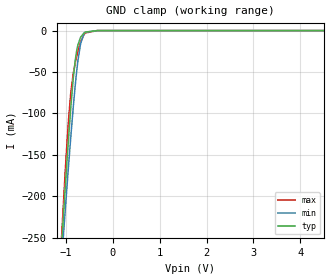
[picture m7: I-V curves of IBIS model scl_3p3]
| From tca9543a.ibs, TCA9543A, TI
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|   scl_3p3 Model
[Model]   scl_3p3
Model_type   Input
Vinl = 0.99
Vinh = 2.31
|   typ   min   max
|   (nom PVT)   (fast PVT)   (slow PVT)
C_comp   7.826e-12   4.224e-12   1.127e-11
[Model spec]
|subparameter
Vinl   0.99   0.9   1.08
Vinh   2.31   2.1   2.52
| Where nom  PVT is Nominal Process, 3.3V, 27C
|   Fast PVT is Strong Process,  3.6V, -40C
|   Slow PVT is Weak Process,   3V, 85C
[Voltage Range]   3.3   3   3.6
|Junction Temperature
[Temperature Range]   27   85   -40
[Power Clamp Reference]   3.3   3   3.6
[GND Clamp Reference]   0   0   0
[GND Clamp]
|   Voltage   I(typ)   I(min)   I(max)
-3.3V     -2.49A     -2.232A    -2.837A
-1.096V   -261.8mA   -280.9mA   -251.9mA
-1.01V    -186mA     -213.8mA   -166mA
-945.6mV  -131.6mA   -164.6mA   -108.9mA
-894.3mV  -91.98mA   -127.3mA   -74.32mA
-843mV    -57.77mA   -92.28mA   -51.81mA
-801mV    -36mA      -66.18mA   -38.98mA
-768mV    -23.75mA   -48.02mA   -30.48mA
-682.8mV  -7.706mA   -15.08mA   -13.24mA
-585mV    -1.752mA   -2.024mA   -2.913mA
-330mV    -5.843uA   -5.757uA   -4.577uA
6.6V      0A         0A         0A
[POWER Clamp]
|   Voltage   I(typ)   I(min)   I(max)
-3.3V     0A         0A         0A
-3.18V    0A         0A         0A
6.6V      0A         0A         0A
